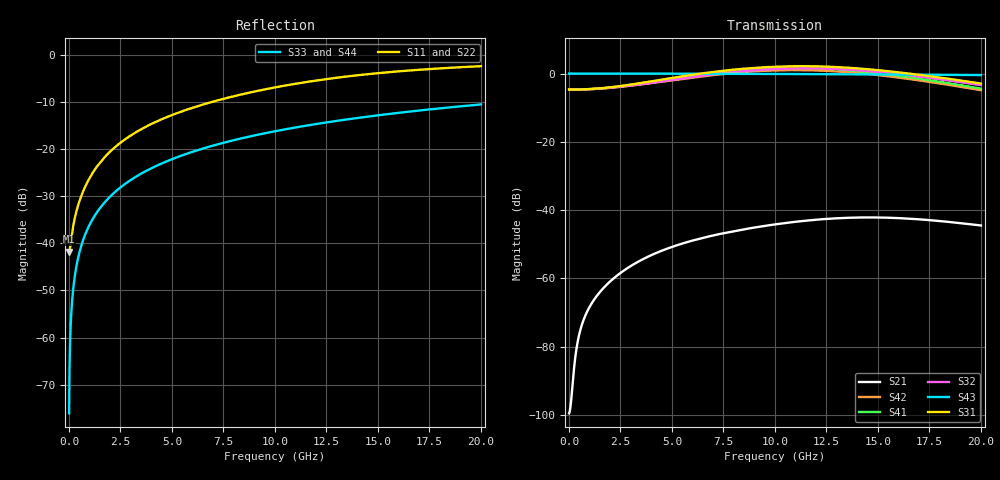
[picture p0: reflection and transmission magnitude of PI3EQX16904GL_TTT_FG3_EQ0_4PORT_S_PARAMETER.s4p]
! NPort=4 DATA=2000 NOISE=0 GROUPDELAY=0 COMPLEX_DATAFORMAT=POLAR
! NumOfBlock=1 NumOfParam=0
! .MODEL Smodel S TSTONEFILE=PI3EQX16904GL_TTT_FG3_EQ0_4PORT_S_PARAMETER.s4p TYPE=S
!  -- The above .MODEL line can be used for the S element in the netlist.
! The s parameter is extracted from the linear redriver, it is not bi-directional; only s(4,1)s(4,2) and s(3,1)s(3,2)
! should be the insertion loss
!Port definition:
!Port1 = input+
!Port2 = input-
!Port3 = output+
!Port4 = output-
# Hz S MA R  50
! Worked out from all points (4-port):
!   2000 points, 10 MHz to 20 GHz, reference 50 ohm
!   strongest paths, dB at 10 MHz, 5.01 GHz, 10.01 GHz, 15.01 GHz, 20 GHz:
!     S31: -4.7, -1.3, 2.0, 1.0, -2.9
!     S43: 0.0, 0.0, -0.1, -0.3, -0.4
!     S32: -4.7, -1.9, 1.4, 0.5, -3.4
!     S41: -4.7, -1.4, 1.6, 0.1, -4.4
!     S42: -4.7, -2.0, 0.9, -0.5, -4.9
!     S21: -99.6, -50.8, -44.2, -42.2, -44.5
!   lowest |S11| = -41.7 dB at 10 MHz (marker M1), VSWR 1.02, Z = 49.2 - j0.0603 ohm
!   |S11| at or under -10 dB: start of sweep to 6.916 GHz
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1e7  0.008182 -175.7  1.049e-05 7.4  0 0.0  0 0.0
     1.049e-05 7.4  0.008182 -175.7  0 0.0  0 0.0
     0.5833 -0.1  0.5833 179.9  0.0001571 -90.0  1 -0.0
     0.5833 179.9  0.5833 -0.1  1 -0.0  0.0001571 -90.0
6.2e8  0.03268 -112.4  0.0002037 112.8  0 0.0  0 0.0
       0.0002037 112.8  0.03268 -112.4  0 0.0  0 0.0
       0.5857 -1.8  0.5846 177.5  0.009738 -90.6  0.9999 -0.6
       0.5856 177.0  0.5845 -3.6  0.9999 -0.6  0.009738 -90.6
2.97e9  0.1383 -101.7  0.00149 92.5  0 0.0  0 0.0
        0.001491 92.5  0.1383 -101.7  0 0.0  0 0.0
        0.6856 -11.4  0.6658 166.0  0.0466 -92.8  0.9988 -2.7
        0.6825 163.3  0.6628 -19.3  0.9988 -2.7  0.0466 -92.8
6.87e9  0.3142 -106.8  0.00416 60.3  0 0.0  0 0.0
        0.004153 60.1  0.3141 -106.9  0 0.0  0 0.0
        1.044 -50.3  0.9636 128.7  0.1072 -96.4  0.9938 -6.2
        1.02 117.5  0.941 -63.5  0.9938 -6.2  0.1072 -96.4
1.035e10  0.4675 -113.9  0.006378 31.7  0 0.0  0 0.0
          0.006357 31.7  0.4665 -114.0  0 0.0  0 0.0
          1.27 -101.8  1.179 78.6  0.1603 -99.6  0.986 -9.2
          1.206 60.2  1.119 -119.4  0.986 -9.2  0.1603 -99.6
1.441e10  0.6224 -123.6  0.007767 -5.3  0 0.0  0 0.0
          0.007786 -5.4  0.6205 -123.6  0 0.0  0 0.0
          1.164 -166.4  1.092 14.6  0.2203 -103.2  0.9734 -12.7
          1.057 -10.6  0.9918 170.3  0.9734 -12.7  0.2203 -103.2
2e10  0.7609 -135.4  0.005946 -44.6  0 0.0  0 0.0
      0.005938 -45.6  0.7593 -135.3  0 0.0  0 0.0
      0.7153 116.8  0.6783 -62.0  0.2986 -108.1  0.9506 -17.4
      0.6023 -95.1  0.5711 86.1  0.9506 -17.4  0.2986 -108.1
